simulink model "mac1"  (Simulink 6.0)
settings: Solver=VariableStepDiscrete  StartTime=0.0  StopTime=20  MaxStep=.1  RelTol=1e-3
undefined symbols (not defined in the file or in its folder): netlist
libraries: xbsIndex_r3 x6

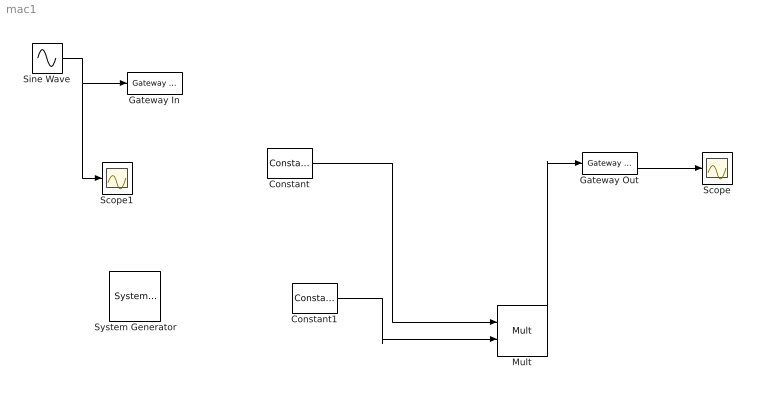
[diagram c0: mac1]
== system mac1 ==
  " System Generator" : xbsIndex_r3/ System Generator  Tag=genX  xilinxfamily=Virtex2  part=xc2v1000  speed=-4  package=bg575  synthesis_tool=XST  directory=./netlist  testbench=off  simulink_period=1  sysclk_period=100  incr_netlist=off  trim_vbits=Everywhere in SubSystem  dbl_ovrd=According to Block Masks  core_generation=According to Block Masks  run_coregen=off  deprecated_control=off  eval_field=0
  Constant : xbsIndex_r3/Constant  const=3  equ=P=C  arith_type=Unsigned  n_bits=2  bin_pt=0  opselect=C  inp2=PCIN>>17  opr=+  inp1=P  carry=CIN  iostate=0  explicit_period=on  period=1  dbl_ovrd=off
  Constant1 : xbsIndex_r3/Constant  const=2  equ=P=C  arith_type=Unsigned  n_bits=2  bin_pt=0  opselect=C  inp2=PCIN>>17  opr=+  inp1=P  carry=CIN  iostate=0  explicit_period=on  period=1  dbl_ovrd=off
  Gateway In : xbsIndex_r3/Gateway In  arith_type="Signed  (2's comp)"  n_bits=8  bin_pt=6  quantization=Truncate  overflow=Wrap  period=1  timing_constraint=None  locs_specified=off  LOCs={}  needs_fixed_name=off  dbl_ovrd=off  show_param=off
  Gateway Out : xbsIndex_r3/Gateway Out  output_type=Double  nbits=8  bin_pt=6  arith_type=Boolean  quantization=Truncate  overflow=Wrap  hdl_port=on  timing_constraint=None  locs_specified=off  LOCs={}  needs_fixed_name=off  show_param=off
  Mult : xbsIndex_r3/Mult  precision=Full  arith_type="Signed  (2's comp)"  n_bits=8  bin_pt=2  quantization=Truncate  overflow=Wrap  latency=3  explicit_period=off  period=1  en=off  dbl_ovrd=off  show_param=off  mult_type=Parallel  oversample=2  use_embedded=off  pipeline=on  use_rpm=on  placement_style=Rectangular Shape  gen_core=off
  Scope : Scope
  Scope1 : Scope
  Sine Wave : Sin  SampleTime=0
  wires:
  Mult/1 -> Gateway Out/1
  Gateway Out/1 -> Scope/1
  Sine Wave/1 -> Gateway In/1, Scope1/1
  Constant/1 -> Mult/1
  Constant1/1 -> Mult/2
